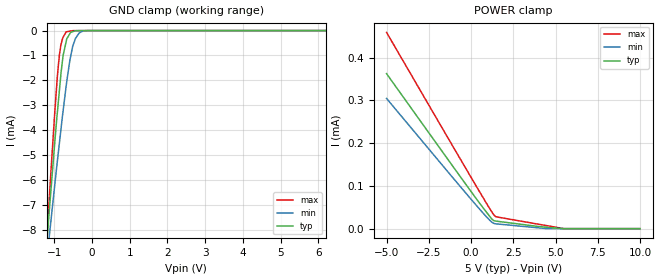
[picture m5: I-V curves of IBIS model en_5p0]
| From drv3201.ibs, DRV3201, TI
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|   en_5p0 Model
[Model]   en_5p0
Model_type   Input
Vinl = 1.5
Vinh = 3.5
|   typ   min   max
|   (nom PVT)   (fast PVT)   (slow PVT)
 C_comp   4.496e-13   4.413e-13   4.851e-13
| Where nom  PVT is Nominal Process, 5V, 27C
|   Fast PVT is Strong Process,  5.5V, -40C
|   Slow PVT is Weak Process,   4.5V, 150C
[Voltage Range]   5   4.5   5.5
[Temperature Range]   27   150   -40
[Power Clamp Reference]   5   4.5   5.5
[GND Clamp Reference]   0   0   0
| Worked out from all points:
|   GND clamp passes 1 mA (typ) near -0.77 V on its own axis
[GND Clamp]
|   Voltage   I(typ)   I(min)   I(max)
-5V       -87.86mA   -68.7mA    -109.7mA
-1.21V    -8.661mA   -9.327mA   -8.562mA
-1.139V   -7.27mA    -8.282mA   -6.781mA
-1.083V   -6.232mA   -7.501mA   -5.439mA
-940.5mV  -3.582mA   -5.485mA   -2.209mA
-869mV    -2.414mA   -4.527mA   -991.1uA
-770mV    -1.001mA   -3.224mA   -265.2uA
-687.5mV  -430.1uA   -2.211mA   -51.29uA
-513mV    -43.17uA   -623.2uA   -3.554uA
-346.5mV  -2.448uA   -104.7uA   -2.389uA
-202.5mV  -1.431uA   -6.568uA   -1.396uA
10V       0A         0A         0A
[POWER Clamp]
|   Voltage   I(typ)   I(min)   I(max)
-5V       362.7uA    304.7uA    459.2uA
500mV     59.84uA    46uA       86.72uA
1.205V    23.67uA    16.07uA    40.68uA
1.441V    17.83uA    11.47uA    28.59uA
4.495V    3.248uA    19.56nA    6.925uA
5.495V    0A         0A         37.91nA
10V       0A         0A         0A
